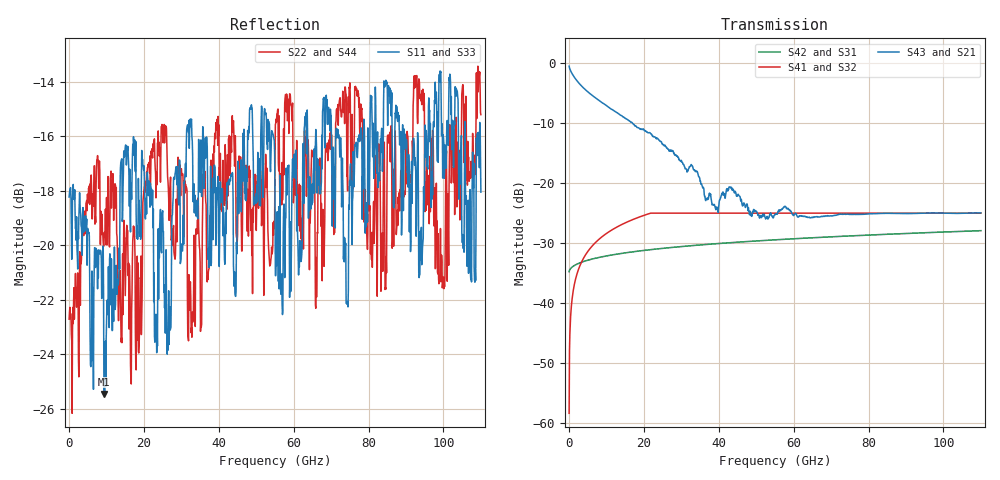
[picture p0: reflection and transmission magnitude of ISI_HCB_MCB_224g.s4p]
! Created with skrf 1.10.0 (http://scikit-rf.org).
# GHz S RI R 50.0
!freq ReS11 ImS11 ReS12 ImS12 ReS13 ImS13
! ReS14 ImS14
! ReS21 ImS21 ReS22 ImS22 ReS23 ImS23
! ReS24 ImS24
! ReS31 ImS31 ReS32 ImS32 ReS33 ImS33
! ReS34 ImS34
! ReS41 ImS41 ReS42 ImS42 ReS43 ImS43
! ReS44 ImS44
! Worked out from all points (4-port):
!   1101 points, 10 MHz to 110 GHz, reference 50 ohm
!   strongest paths, dB at 10 MHz, 27.51 GHz, 55.01 GHz, 82.5 GHz, 110 GHz:
!     S43: -0.5, -14.6, -25.3, -25.1, -25.0
!     S21: -0.5, -14.5, -25.2, -25.2, -25.1
!     S41: -58.4, -25.0, -25.0, -25.0, -25.0
!     S32: -58.4, -25.0, -25.0, -25.0, -25.0
!     S42: -34.8, -30.8, -29.5, -28.6, -28.0
!     S31: -34.8, -30.8, -29.5, -28.6, -28.0
!   lowest |S11| = -25.5 dB at 9.309 GHz (marker M1), VSWR 1.11, Z = 54.4 - j3.43 ohm
!   |S11| at or under -10 dB: start of sweep to end of sweep
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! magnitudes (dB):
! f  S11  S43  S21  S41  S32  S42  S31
! 10 MHz  -18.2  -0.5  -0.5  -58.4  -58.4  -34.8  -34.8
! 1.81 GHz  -19.3  -2.7  -2.7  -35.8  -35.8  -33.6  -33.6
! 9.309 GHz  -25.5  -6.8  -6.9  -28.7  -28.7  -32.3  -32.3
! 39.41 GHz  -18.4  -24.1  -24.1  -25.0  -25.0  -30.1  -30.1
! 92.4 GHz  -16.8  -25.1  -25.0  -25.0  -25.0  -28.4  -28.4
! 99.8 GHz  -17.5  -25.0  -25.0  -25.0  -25.0  -28.2  -28.2
! 110 GHz  -18.0  -25.0  -25.1  -25.0  -25.0  -28.0  -28.0
